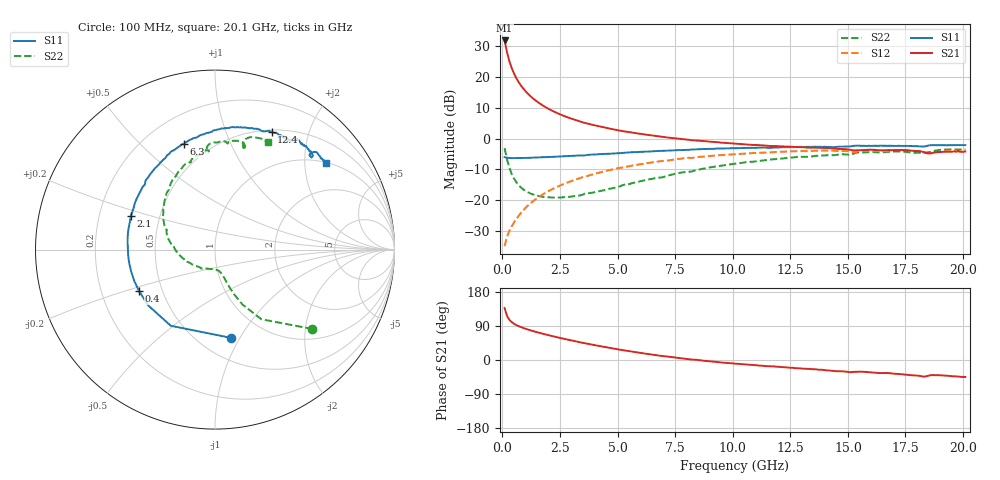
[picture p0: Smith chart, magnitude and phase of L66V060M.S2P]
!  Infineon Technologies AG
! BFR380L3 , PF131585-7, No.6, Th 09.10.01, soldered on pcb-board, measured with PP GSG850
!  Vce=6.0 V,  Ic=60.0 mA
! Common Emitter S-Parameters:  15. November 2001
#  GHz  S  MA  R  50
! f  S11  S21  S12  S22
! GHz  Mag  Ang  Mag  Ang  Mag  Ang  Mag  Ang
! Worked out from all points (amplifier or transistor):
!   201 points, 100 MHz to 20.1 GHz, reference 50 ohm
!   highest |S21| = 31.9 dB at 100 MHz (marker M1)
!   |S21| within 3 dB of that: start of sweep to 181.7 MHz
!   unconditionally stable (mu >= 1): 871.9 MHz to 4.263 GHz; 18.24 GHz to 18.6 GHz
!   at 3.4 GHz: K = 1.03, MAG = 8.1 dB, |S12| = -12.7 dB
!   at 10.1 GHz: K = 0.94, MSG = 1.7 dB, |S12| = -5.0 dB
!   at 20.1 GHz: K = 0.99, MSG = -0.1 dB, |S12| = -4.0 dB
!   S11 on the Smith chart (normalised r, x): 100 MHz: 0.70, -0.91; 400 MHz: 0.37, -0.22; 2.1 GHz: 0.34, +0.17; 6.3 GHz: 0.36, +0.68; 12.4 GHz: 0.52, +1.46; 20.1 GHz: 1.02, +2.55
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0.1  0.499 -79.9  39.19 137.3  0.01794 59.8  0.7004 -39.2
0.2  0.4907 -120.1  25.67 116.8  0.02513 56.6  0.4662 -56.3
0.3  0.4849 -139.9  18.42 106.7  0.03144 58.1  0.3419 -63.4
0.4  0.4822 -151.3  14.23 100.4  0.03701 60.4  0.2713 -66.8
0.5  0.4826 -159.3  11.55 95.9  0.0429 62.7  0.2273 -68.8
0.6  0.483 -165.2  9.707 92.4  0.04917 64.3  0.1983 -70.1
0.7  0.4835 -169.7  8.372 89.5  0.05523 65.7  0.1772 -71.2
0.9  0.4849 -176.9  6.561 84.7  0.06817 67.3  0.1507 -72.9
1.1  0.4864 177.7  5.407 80.6  0.08112 68.2  0.1354 -75.3
1.4  0.4924 170.8  4.283 75.1  0.1006 68.4  0.1217 -79.3
1.7  0.4963 164.9  3.557 70.2  0.1204 67.8  0.1145 -84.5
2.1  0.5055 158.0  2.914 64.1  0.1466 66.4  0.111 -92.3
2.7  0.5176 148.8  2.314 55.6  0.1856 63.6  0.1118 -105.6
3.5  0.5324 137.4  1.834 45.2  0.2372 58.9  0.1235 -122.1
4.8  0.5732 122.0  1.419 30.4  0.3168 50.7  0.1569 -151.2
6.3  0.6148 106.4  1.15 16.0  0.4017 40.4  0.2153 -177.4
6.8  0.6296 101.7  1.084 11.6  0.4277 36.7  0.2322 174.9
10.1  0.6986 76.9  0.8259 -9.6  0.5595 14.5  0.3915 135.8
12.4  0.7286 64.3  0.7429 -19.8  0.6192 -0.5  0.4855 113.2
13.5  0.7355 59.2  0.7152 -24.4  0.6324 -7.2  0.5179 104.5
16.8  0.7651 47.1  0.6522 -34.8  0.638 -23.9  0.6125 81.2
20.1  0.7839 37.9  0.6168 -44.9  0.6287 -38.0  0.6707 63.8
